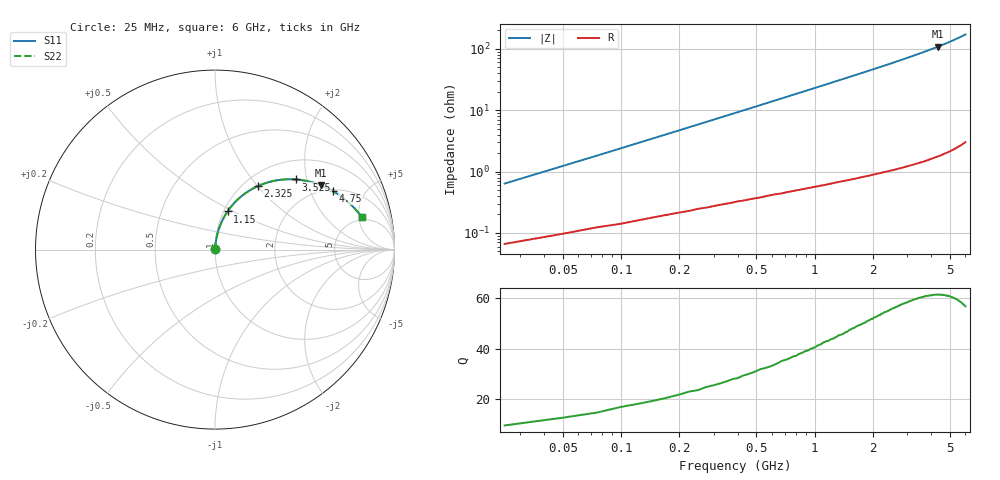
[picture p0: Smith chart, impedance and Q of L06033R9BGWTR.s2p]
!	AVX Thin Film Operation
!	Date:	March	2003
!	Description: Accu-L® Series Thin Film SMD RF Inductors
!	Part Number: L06033R9BGWTR
!	25MHz-6GHz
!	Serial	Measurements
#	mhz	S	db	R	50
!	S11	S11	S21	S21	S12	S12	S22	S22
!	dB	Phase	dB	Phase	dB	Phase	dB	Phase
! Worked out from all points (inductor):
!   240 points, 25 MHz to 6 GHz, reference 50 ohm
!   read as one part in series: L = 3.85 nH near 50 MHz
!   highest Q = 61.3 at 4.325 GHz (marker M1), where L = 3.97 nH
!   S11 on the Smith chart (normalised r, x): 25 MHz: 1.00, +0.01; 1.15 GHz: 1.04, +0.47; 2.325 GHz: 1.16, +1.00; 3.525 GHz: 1.42, +1.72; 4.75 GHz: 2.06, +2.91; 6 GHz: 4.51, +5.49
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25  -44.93 83.0  -0.01 -0.4  -0.01 -0.4  -44.93 83.0
50  -39.25 84.1  -0.01 -0.8  -0.01 -0.8  -39.25 84.1
75  -35.90 84.5  -0.01 -1.2  -0.01 -1.2  -35.90 84.5
100  -33.50 84.6  -0.01 -1.5  -0.01 -1.5  -33.50 84.6
125  -31.64 84.5  -0.02 -1.9  -0.02 -1.9  -31.64 84.5
175  -28.82 84.2  -0.02 -2.6  -0.02 -2.6  -28.82 84.2
275  -25.01 83.2  -0.04 -4.1  -0.04 -4.1  -25.01 83.2
400  -21.85 81.8  -0.06 -5.9  -0.06 -5.9  -21.85 81.8
575  -18.79 79.6  -0.09 -8.5  -0.09 -8.5  -18.79 79.6
775  -16.28 76.9  -0.14 -11.3  -0.14 -11.3  -16.28 76.9
1025  -13.95 73.5  -0.23 -14.9  -0.23 -14.9  -13.95 73.5
1150  -13.00 71.8  -0.28 -16.6  -0.28 -16.6  -13.00 71.8
1550  -10.57 66.4  -0.46 -22.2  -0.46 -22.2  -10.57 66.4
2025  -8.46 60.0  -0.74 -28.7  -0.74 -28.7  -8.46 60.0
2325  -7.41 56.1  -0.96 -32.7  -0.96 -32.7  -7.41 56.1
3025  -5.50 47.1  -1.54 -41.8  -1.54 -41.8  -5.50 47.1
3525  -4.48 40.9  -2.04 -48.1  -2.04 -48.1  -4.48 40.9
4025  -3.64 34.8  -2.60 -54.1  -2.60 -54.1  -3.64 34.8
4325  -3.22 31.3  -2.97 -57.7  -2.97 -57.7  -3.22 31.3
4750  -2.69 26.4  -3.53 -62.6  -3.53 -62.6  -2.69 26.4
5025  -2.39 23.3  -3.92 -65.7  -3.92 -65.7  -2.39 23.3
6000  -1.54 12.5  -5.53 -76.4  -5.53 -76.4  -1.54 12.5
